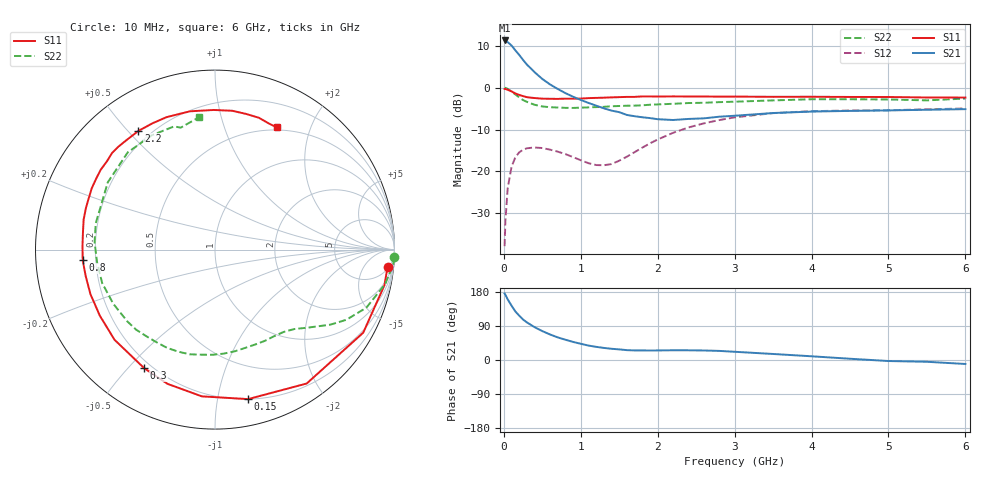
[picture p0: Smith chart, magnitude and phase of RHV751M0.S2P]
! SIEMENS Small Signal Semiconductors
! BFR106
! Si NPN RF Bipolar Junction Transistor in SOT23
! VCE = 0.75 V  IC = 1 mA
! Common Emitter S-Parameters:  August  1996
# GHz  S  MA  R  50
!  f  S11  S21  S12  S22
! GHz  MAG  ANG  MAG  ANG  MAG  ANG  MAG  ANG
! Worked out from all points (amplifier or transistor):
!   36 points, 10 MHz to 6 GHz, reference 50 ohm
!   highest |S21| = 11.3 dB at 10 MHz (marker M1)
!   |S21| within 3 dB of that: start of sweep to 178.7 MHz
!   unconditionally stable (mu >= 1): 827.8 MHz to end of sweep
!   at 250 MHz: K = 0.31, MSG = 10.7 dB, |S12| = -14.8 dB
!   at 1.4 GHz: K = 1.62, MAG = 1.8 dB, |S12| = -18.3 dB
!   at 6 GHz: K = 1.02, MAG = -1.0 dB, |S12| = -5.0 dB
!   S11 on the Smith chart (normalised r, x): 10 MHz: 6, -17; 150 MHz: 0.20, -1.23; 300 MHz: 0.17, -0.56; 800 MHz: 0.15, -0.04; 2.2 GHz: 0.15, +0.53; 6 GHz: 0.47, +1.52
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0.01  0.9662 -5.9  3.678 175.5  0.0127 86.7  0.9977 -2.5
0.02  0.9646 -11.9  3.644 172.2  0.0253 82.4  0.9967 -4.7
0.05  0.9467 -29.3  3.517 160.0  0.0623 72.4  0.968 -11.4
0.1  0.9042 -55.6  3.202 143.5  0.1132 58.1  0.9032 -21.0
0.15  0.8532 -77.5  2.798 128.0  0.1474 45.8  0.8299 -28.1
0.2  0.821 -95.1  2.468 117.1  0.1686 36.9  0.7673 -33.0
0.25  0.7934 -109.5  2.151 106.8  0.1813 29.4  0.7114 -37.0
0.3  0.7696 -120.8  1.893 99.2  0.1887 24.3  0.6773 -39.9
0.4  0.7522 -138.1  1.533 86.6  0.1926 16.0  0.625 -45.1
0.5  0.7398 -150.2  1.273 76.3  0.1897 10.4  0.5972 -50.2
0.6  0.737 -160.4  1.096 67.4  0.1816 6.7  0.5845 -55.5
0.8  0.7394 -175.4  0.862 53.5  0.1606 3.8  0.5744 -66.8
1.1  0.7508 167.1  0.658 38.1  0.1251 12.2  0.5815 -85.1
1.4  0.7669 153.6  0.532 29.6  0.122 36.5  0.6002 -103.6
1.8  0.7865 136.8  0.443 25.3  0.1919 55.4  0.6157 -128.3
2.2  0.7871 122.9  0.411 25.7  0.2886 53.4  0.6422 -152.0
2.8  0.7817 105.0  0.45 24.0  0.4099 40.3  0.6722 176.4
3.5  0.778 90.5  0.498 15.9  0.4965 24.3  0.7052 147.9
4.5  0.7755 77.2  0.528 3.3  0.5336 6.4  0.7278 119.0
5  0.7742 71.6  0.535 -2.7  0.5374 -0.2  0.7233 108.4
5.5  0.7639 66.8  0.545 -4.7  0.5513 -3.3  0.7057 105.7
6  0.7628 63.2  0.554 -10.5  0.5647 -9.9  0.742 97.0
